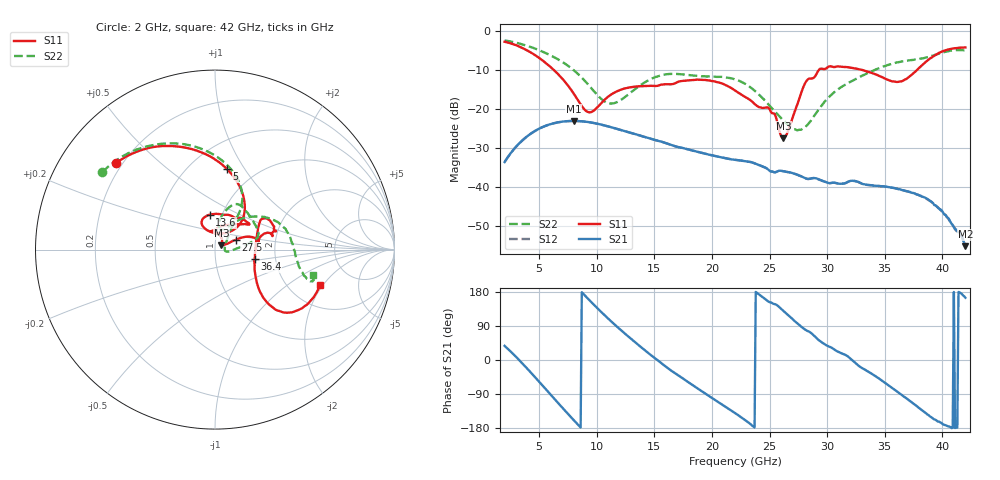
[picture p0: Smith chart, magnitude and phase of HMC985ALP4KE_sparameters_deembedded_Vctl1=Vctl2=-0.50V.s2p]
!s2p File: Measurements: S11, S21, S12, S22
# GHz S dB R 50.0
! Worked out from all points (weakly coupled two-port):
!   401 points, 2 GHz to 42 GHz, reference 50 ohm
!   highest |S21| = -23.00 dB at 8 GHz (marker M1); lowest = -55.1 dB at 42 GHz (marker M2)
!   lowest |S11| = -27.4 dB at 26.2 GHz (marker M3), VSWR 1.09, Z = 53.6 + j2.52 ohm
!   |S11| at or under -10 dB: 6.294 GHz to 29.26 GHz (22.97 GHz wide, 129 % of centre); 33.12 GHz to 37.78 GHz (4.655 GHz wide, 13.1 % of centre)
!   |S22| runs from -25.4 to -2.4 dB; largest |S21 - S12| = 0.0002
!   S11 on the Smith chart (normalised r, x): 2 GHz: 0.17, +0.36; 5 GHz: 0.74, +0.84; 13.6 GHz: 0.88, +0.35; 27.5 GHz: 1.25, +0.14; 36.4 GHz: 1.55, -0.17; 42 GHz: 2.95, -1.89
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2  -2.69 139.0  -33.56 37.3  -33.55 37.3  -2.37 145.5
3.4  -4.10 112.4  -28.39 -4.5  -28.39 -4.4  -3.26 123.1
5  -6.85 81.7  -24.98 -57.4  -24.99 -57.4  -4.86 98.5
8  -16.00 46.3  -23.00 -158.7  -23.01 -158.7  -9.99 61.3
8.7  -19.21 57.4  -23.10 178.7  -23.10 178.7  -11.91 57.1
9.5  -20.75 88.8  -23.40 153.5  -23.40 153.5  -14.50 56.1
11.1  -16.54 117.6  -24.50 106.1  -24.50 106.1  -18.52 71.8
13.6  -14.13 98.7  -26.62 39.9  -26.63 39.9  -14.24 78.2
15.4  -13.89 73.8  -28.17 -3.3  -28.18 -3.3  -11.45 68.3
19.4  -12.50 36.4  -31.41 -88.1  -31.41 -88.2  -11.58 34.9
22  -15.16 53.7  -32.98 -139.9  -32.98 -139.8  -12.35 14.9
24.9  -19.61 96.7  -35.51 154.2  -35.50 154.3  -18.75 1.8
26.2  -27.44 33.6  -35.90 129.2  -35.90 129.2  -22.93 -9.0
27.5  -17.96 25.4  -36.94 94.3  -36.90 94.1  -25.34 1.4
28.1  -13.24 18.7  -37.67 79.9  -37.66 79.8  -24.58 18.8
28.7  -12.10 11.3  -37.71 68.9  -37.69 68.7  -22.45 33.8
31  -9.05 21.9  -39.09 21.1  -39.10 21.3  -14.77 53.3
33.3  -10.16 33.1  -39.32 -25.7  -39.30 -25.7  -11.06 41.0
35.4  -12.60 11.6  -40.00 -68.4  -40.00 -68.6  -8.56 25.2
36.4  -12.89 -13.6  -40.61 -90.5  -40.66 -90.8  -7.79 16.8
39.5  -5.94 -43.2  -44.92 -159.7  -44.85 -159.3  -5.91 -14.9
42  -4.15 -18.5  -55.13 164.3  -54.85 166.0  -4.94 -14.3
